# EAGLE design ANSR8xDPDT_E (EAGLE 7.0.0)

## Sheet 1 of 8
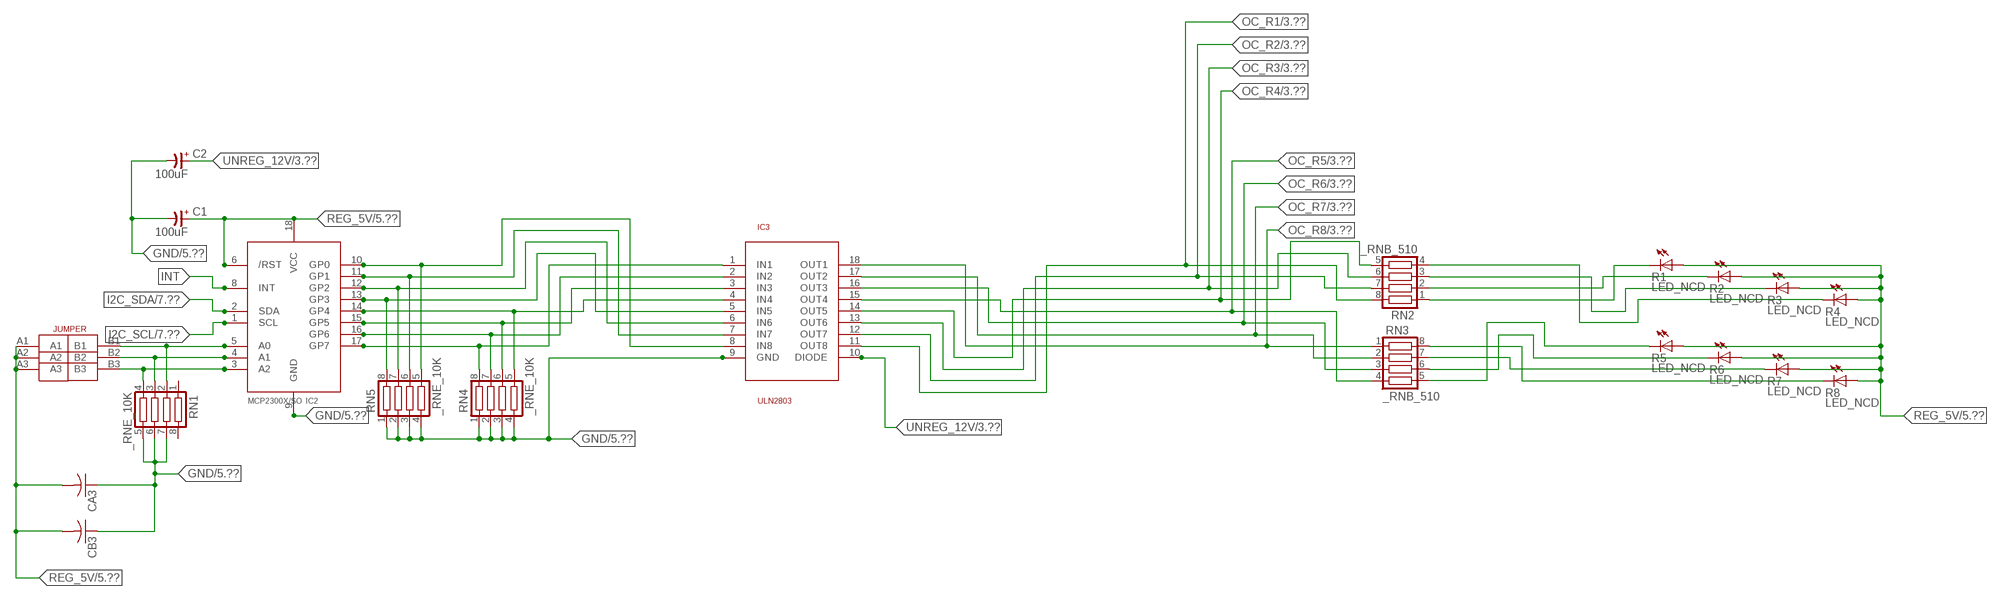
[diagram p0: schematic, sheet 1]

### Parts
C1  100uF  CP-E-025X060  [E-025X060]
C2  100uF  CP-E-025X060  [E-025X060]
CA3  CC1206KRX7R9BB104C1206K  [CC1206KRX7R9BB104]
CB3  TMK316F106ZL-TC1206K  [TMK316F106ZL-T]
IC2  MCP2300X/SO  [SO18W]
IC3  ULN2803  [SO18L]
R1  LED_NCD  [CHIPLED_0603]
R2  LED_NCD  [CHIPLED_0603]
R3  LED_NCD  [CHIPLED_0603]
R4  LED_NCD  [CHIPLED_0603]
R5  LED_NCD  [CHIPLED_0603]
R6  LED_NCD  [CHIPLED_0603]
R7  LED_NCD  [CHIPLED_0603]
R8  LED_NCD  [CHIPLED_0603]
RN1  _RNE_10K  [RNE]
RN2  _RNB_510  [RNB]
RN3  _RNB_510  [RNB]
RN4  _RNE_10K  [RNE]
RN5  _RNE_10K  [RNE]
U$18  JUMPER_3X2  [JUMPER_3X2]

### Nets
GND: C1.- C2.- CA3.1 CB3.1 IC2.9(GND) IC3.9(GND) RN1.5 RN1.6 RN1.7 RN4.1 RN4.2 RN4.3 RN4.4 RN5.1 RN5.2 RN5.3 RN5.4 ; also sheet 5,6,7,8
GP4: IC2.14(GP4) IC3.4(IN4) RN4.5
GP6: IC2.16(GP6) IC3.2(IN2) RN4.7
I2C_SCL: IC2.1(SCL) ; also sheet 7,8
I2C_SDA: IC2.2(SDA) ; also sheet 7,8
INT: IC2.8(INT)
N$6: IC2.5(A0) RN1.2 U$18.B1
N$7: IC2.4(A1) RN1.3 U$18.B2
N$8: IC2.3(A2) RN1.4 U$18.B3
N$20: R1.C RN2.1
N$21: IC2.12(GP2) IC3.6(IN6) RN5.7
N$22: IC2.11(GP1) IC3.7(IN7) RN5.6
N$23: IC2.10(GP0) IC3.8(IN8) RN5.5
N$29: R2.C RN2.2
N$30: R3.C RN2.3
N$31: R4.C RN2.4
N$32: R8.C RN3.8
N$81: R7.C RN3.7
N$82: R6.C RN3.6
N$83: R5.C RN3.5
N$89: IC2.13(GP3) IC3.5(IN5) RN5.8
N$93: IC2.15(GP5) IC3.3(IN3) RN4.6
N$94: IC2.17(GP7) IC3.1(IN1) RN4.8
OC_R1: IC3.11(OUT8) RN2.8 ; also sheet 3
OC_R2: IC3.12(OUT7) RN2.7 ; also sheet 3
OC_R3: IC3.13(OUT6) RN2.6 ; also sheet 3
OC_R4: IC3.14(OUT5) RN2.5 ; also sheet 3
OC_R5: IC3.15(OUT4) RN3.4 ; also sheet 3
OC_R6: IC3.16(OUT3) RN3.3 ; also sheet 3
OC_R7: IC3.17(OUT2) RN3.2 ; also sheet 3
OC_R8: IC3.18(OUT1) RN3.1 ; also sheet 3
REG_5V: C1.+ CA3.2 CB3.2 IC2.6(/RST) IC2.18(VCC) R1.A R2.A R3.A R4.A R5.A R6.A R7.A R8.A U$18.A1 U$18.A2 U$18.A3 ; also sheet 5,6,7,8
UNREG_12V: C2.+ IC3.10(DIODE) ; also sheet 3,5
Unconnected: RN1.1 RN1.8

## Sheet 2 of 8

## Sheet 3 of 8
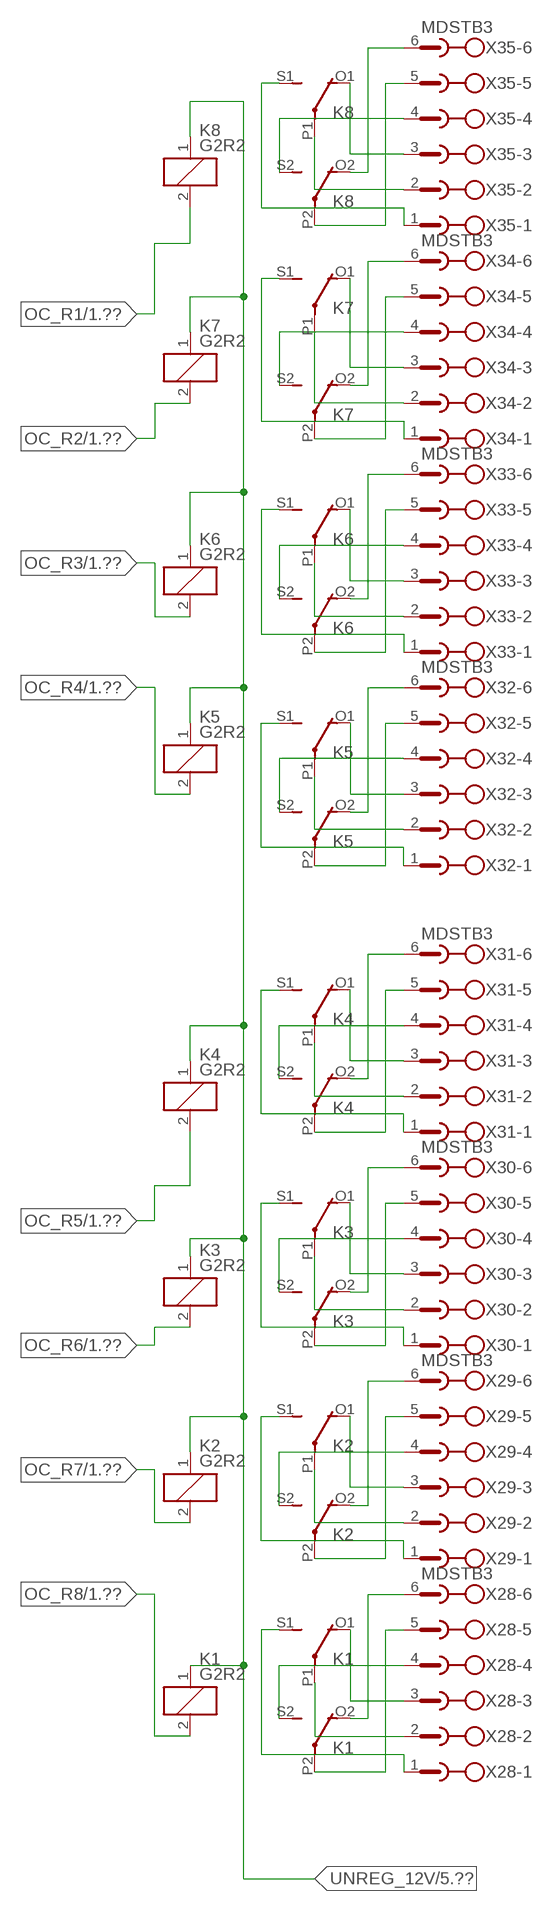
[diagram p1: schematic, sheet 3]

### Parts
K1  G2R2  [G2R2]
K2  G2R2  [G2R2]
K3  G2R2  [G2R2]
K4  G2R2  [G2R2]
K5  G2R2  [G2R2]
K6  G2R2  [G2R2]
K7  G2R2  [G2R2]
K8  G2R2  [G2R2]
X28  MDSTB3  [MDSTB3]
X29  MDSTB3  [MDSTB3]
X30  MDSTB3  [MDSTB3]
X31  MDSTB3  [MDSTB3]
X32  MDSTB3  [MDSTB3]
X33  MDSTB3  [MDSTB3]
X34  MDSTB3  [MDSTB3]
X35  MDSTB3  [MDSTB3]

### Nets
N$84: K1.P2(3:COM) X28.5
N$85: K1.O2(3:NC) X28.6
N$86: K1.S2(3:NO) X28.4
N$87: K1.P1(2:COM) X28.2
N$88: K1.O1(2:NC) X28.3
N$90: K1.S1(2:NO) X28.1
N$91: K2.P2(3:COM) X29.5
N$92: K2.O2(3:NC) X29.6
N$95: K2.S2(3:NO) X29.4
N$96: K2.S1(2:NO) X29.1
N$97: K2.P1(2:COM) X29.2
N$98: K2.O1(2:NC) X29.3
N$99: K3.P2(3:COM) X30.5
N$100: K3.O2(3:NC) X30.6
N$101: K4.P2(3:COM) X31.5
N$102: K4.O2(3:NC) X31.6
N$103: K3.S2(3:NO) X30.4
N$104: K4.S2(3:NO) X31.4
N$105: K3.O1(2:NC) X30.3
N$106: K4.O1(2:NC) X31.3
N$107: K4.P1(2:COM) X31.2
N$108: K3.P1(2:COM) X30.2
N$109: K3.S1(2:NO) X30.1
N$110: K4.S1(2:NO) X31.1
N$111: K5.O2(3:NC) X32.6
N$112: K5.P2(3:COM) X32.5
N$113: K5.S2(3:NO) X32.4
N$114: K5.P1(2:COM) X32.2
N$115: K5.S1(2:NO) X32.1
N$116: K5.O1(2:NC) X32.3
N$117: K6.P2(3:COM) X33.5
N$118: K6.O2(3:NC) X33.6
N$119: K6.P1(2:COM) X33.2
N$120: K6.S1(2:NO) X33.1
N$121: K7.P1(2:COM) X34.2
N$122: K8.P1(2:COM) X35.2
N$316: K8.P2(3:COM) X35.5
N$317: K8.O2(3:NC) X35.6
N$318: K6.O1(2:NC) X33.3
N$319: K8.O1(2:NC) X35.3
N$320: K7.O1(2:NC) X34.3
N$321: K7.O2(3:NC) X34.6
N$322: K7.P2(3:COM) X34.5
N$323: K6.S2(3:NO) X33.4
N$324: K7.S2(3:NO) X34.4
N$325: K7.S1(2:NO) X34.1
N$326: K8.S1(2:NO) X35.1
N$327: K8.S2(3:NO) X35.4
OC_R1: K8.2(1:C2) ; also sheet 1
OC_R2: K7.2(1:C2) ; also sheet 1
OC_R3: K6.2(1:C2) ; also sheet 1
OC_R4: K5.2(1:C2) ; also sheet 1
OC_R5: K4.2(1:C2) ; also sheet 1
OC_R6: K3.2(1:C2) ; also sheet 1
OC_R7: K2.2(1:C2) ; also sheet 1
OC_R8: K1.2(1:C2) ; also sheet 1
UNREG_12V: K1.1(1:C1) K2.1(1:C1) K3.1(1:C1) K4.1(1:C1) K5.1(1:C1) K6.1(1:C1) K7.1(1:C1) K8.1(1:C1) ; also sheet 1,5

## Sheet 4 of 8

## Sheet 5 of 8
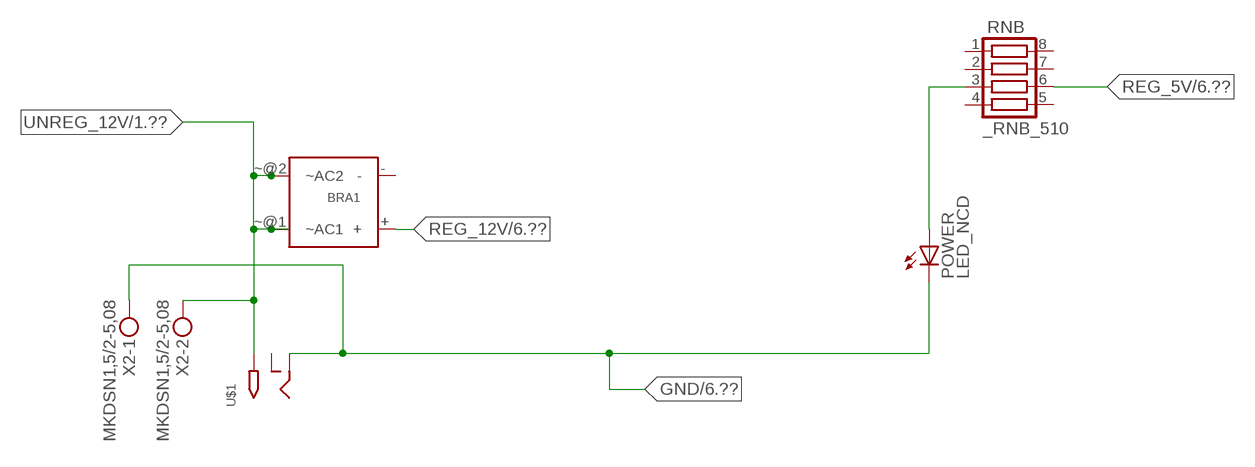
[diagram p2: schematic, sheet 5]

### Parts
BRA1  MB2S_  [MB2S]
POWER  LED_NCD  [CHIPLED_0603]
RNB  _RNB_510  [RNB]
U$1  2.1MMJACK  [PJ-102A]
X2  MKDSN1,5/2-5,08  [MKDSN1,5/2-5,08]

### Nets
GND: POWER.C U$1.RING X2.1 ; also sheet 1,6,7,8
N$2: POWER.A RNB.3
REG_5V: RNB.6 ; also sheet 1,6,7,8
REG_12V: BRA1.+ ; also sheet 6
UNREG_12V: BRA1.~@1(~AC1) BRA1.~@2(~AC2) U$1.TIP X2.2 ; also sheet 1,3
Unconnected: BRA1.- RNB.1 RNB.2 RNB.4 RNB.5 RNB.7 RNB.8 U$1.RING_SW

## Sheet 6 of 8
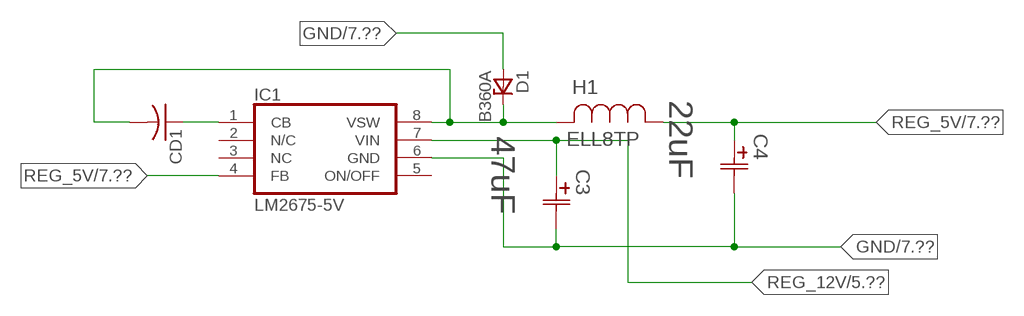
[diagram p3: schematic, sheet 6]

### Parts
C3  47uF  490-5463-6-NDCAP  [C2917(7343)-Y]
C4  22uF  490-5463-6-NDCAP  [C2917(7343)-Y]
CD1  _CD_10NF_50VC1206K  [_CD_10NF_50V]
D1  B360A  [DO214AC_ZENER]
H1  ELL8TP  [IND_ELL8TP]
IC1  LM2675-5V  LM2675  [SO-8]

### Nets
GND: C3.2(C2) C4.2(C2) D1.A IC1.6(GND) ; also sheet 1,5,7,8
N$1: CD1.2 D1.C H1.2 IC1.8(VSW)
N$3: CD1.1 IC1.1(CB)
REG_5V: C4.1(C1) H1.1 IC1.4(FB) ; also sheet 1,5,7,8
REG_12V: C3.1(C1) IC1.7(VIN) ; also sheet 5
Unconnected: IC1.2(N/C) IC1.5(ON/OFF)

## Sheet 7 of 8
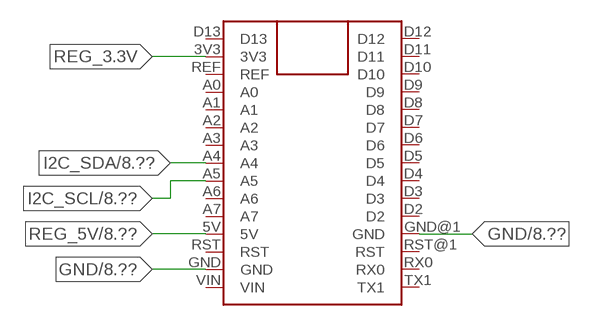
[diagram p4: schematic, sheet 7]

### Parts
FOR_NANO  ARDUINO_NANO  [ARDUINO_NANO]

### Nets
GND: FOR_NANO.GND FOR_NANO.GND@1(GND) ; also sheet 1,5,6,8
I2C_SCL: FOR_NANO.A5 ; also sheet 1,8
I2C_SDA: FOR_NANO.A4 ; also sheet 1,8
REG_3.3V: FOR_NANO.3V3
REG_5V: FOR_NANO.5V ; also sheet 1,5,6,8
Unconnected: FOR_NANO.A0 FOR_NANO.A1 FOR_NANO.A2 FOR_NANO.A3 FOR_NANO.A6 FOR_NANO.A7 FOR_NANO.D2 FOR_NANO.D3 FOR_NANO.D4 FOR_NANO.D5 FOR_NANO.D6 FOR_NANO.D7 FOR_NANO.D8 FOR_NANO.D9 FOR_NANO.D10 FOR_NANO.D11 FOR_NANO.D12 FOR_NANO.D13 FOR_NANO.REF FOR_NANO.RST FOR_NANO.RST@1(RST) FOR_NANO.RX0 FOR_NANO.TX1 FOR_NANO.VIN

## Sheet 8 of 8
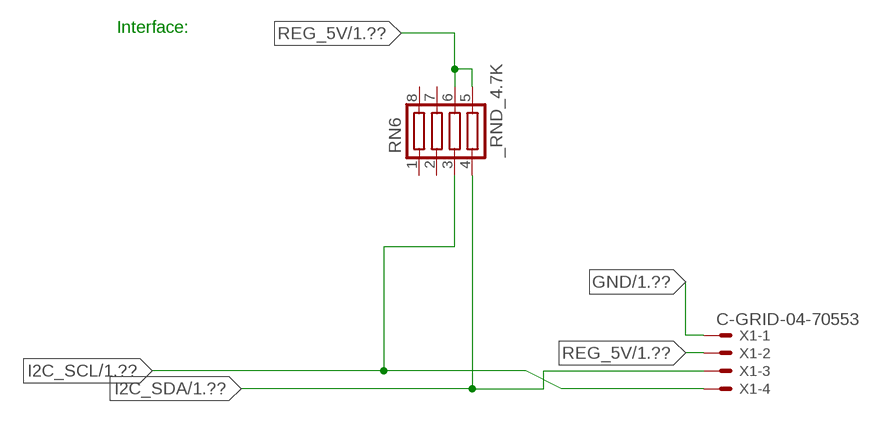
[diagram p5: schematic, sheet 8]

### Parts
RN6  _RND_4.7K  [RND]
X1  C-GRID-04-70553  [70553-04]

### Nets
GND: X1.1 ; also sheet 1,5,6,7
I2C_SCL: RN6.3 X1.4 ; also sheet 1,7
I2C_SDA: RN6.4 X1.3 ; also sheet 1,7
REG_5V: RN6.5 RN6.6 X1.2 ; also sheet 1,5,6,7
Unconnected: RN6.1 RN6.2 RN6.7 RN6.8

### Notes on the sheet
- Interface:

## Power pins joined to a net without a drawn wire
NC: IC1.3(NC)

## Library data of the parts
BRA1 = NCD_ULTIMATE_LIBRARY:MB2S: Bridge Rectifier BRA MB2S 200V 500ma Digikey MB2S-TPMSTR-ND/MB2S-TP
C1 C2 = NCD_ULTIMATE_LIBRARY:CP-: Capacitors All Kinds POLARIZED CAP
C3 C4 = NCD_ULTIMATE_bhaskar:490-5463-6-ND: NCD CAP
CA3 = NCD_ULTIMATE_LIBRARY:CC1206KRX7R9BB104: Capacitor CA .1uF 50V SMT C1206K CC1206KRX7R9BB104
CB3 = NCD_ULTIMATE_LIBRARY:TMK316F106ZL-T: Capacitor CB 10uF SMT 1206 TMK316F106ZL-T
CD1 = NCD_ULTIMATE_LIBRARY:_CD_10NF_50V: Capacitor 10nF SMT
D1 = NCD_ULTIMATE_bhaskar:B360A: NCD DIODE B350A/B360A
FOR_NANO = NCD_ULTIMATE_CONNECTORS:ARDUINO_NANO
H1 = NCD_ULTIMATE_bhaskar:ELL8TP: NCD coil
IC1 = NCD_ULTIMATE_bhaskar:LM2675: LM2675 NCD http://www.ti.com/lit/ds/symlink/lm2675.pdf
IC2 = NCD_ULTIMATE_LIBRARY:MCP2300X: Semiconductor Port Expander I/O 8-Bit I2C MCP23008 Inexpensive i2c i/o expander - 8 general purpose i/o pins with optional pullups
IC3 = NCD_ULTIMATE_LIBRARY:ULN2803: Semiconductor 8 O.C. N-Channel Transistor Driver Digikey ULN2803AFWGCELTR-ND/ULN2803AFWG,C,EL
K1-K8 = NCD_ULTIMATE_LIBRARY:G2R2: RELAY 2 x switch, Omron
POWER = NCD_ULTIMATE_bhaskar:LED_NCD
R1-R8 = NCD_ULTIMATE_LIBRARY:LED_NCD: LED Digikey 754-1132-2-ND/APT2012SRCPRV
RN1 RN4 RN5 = NCD_ULTIMATE_LIBRARY:_RNE_10K: Resistor Array RNE SMT 10K x 4 Single Resistor Source: http://www.ctscorp.com/components/Datasheets/CTSChipArrayDs.pdf Digikey 742C083103JPTR-ND/742C083103JP; OC_FARNELL: unknown; OC_NEWARK: unknown
RN2 RN3 RNB = NCD_ULTIMATE_LIBRARY:_RNB_510: Resistor Array RNB SMT 510 x 4 Single Resistor Source: http://www.ctscorp.com/components/Datasheets/CTSChipArrayDs.pdf Digikey 742C083511JPTR-ND/ 742C083511JP; OC_FARNELL: unknown; OC_NEWARK: unknown
RN6 = NCD_ULTIMATE_LIBRARY:_RND_4.7K: Resistor Array RND SMT 4.7K x 4 Single Resistor Source: http://www.ctscorp.com/components/Datasheets/CTSChipArrayDs.pdf Digikey 742C083472JPTR-ND/742C083472JP; OC_FARNELL: unknown; OC_NEWARK: unknown
U$1 = NCD_ULTIMATE_CONNECTORS:2.1MMJACK: 2.1mm x 5.5mm DC jack with internal switch. Digikey part #PJ-102A, 4UCON part #05537 By microbuilder.eu
U$18 = NCD_ULTIMATE_CONNECTORS:JUMPER_3X2
X1 = NCD_ULTIMATE_CONNECTORS:C-GRID-04: CONNECTOR 4-Pos I2C wire to board 2.54 mm (0.100") pitch header Digikey WM1342-ND/0015912045; OC_FARNELL: unknown; OC_NEWARK: unknown
X2 = NCD_ULTIMATE_CONNECTORS:MKDSN1,5/2-5,08: MKDSN 1,5/ 2-5,08 Printklemme
X28-X35 = NCD_ULTIMATE_LIBRARY:MDSTB3: PHOENIX

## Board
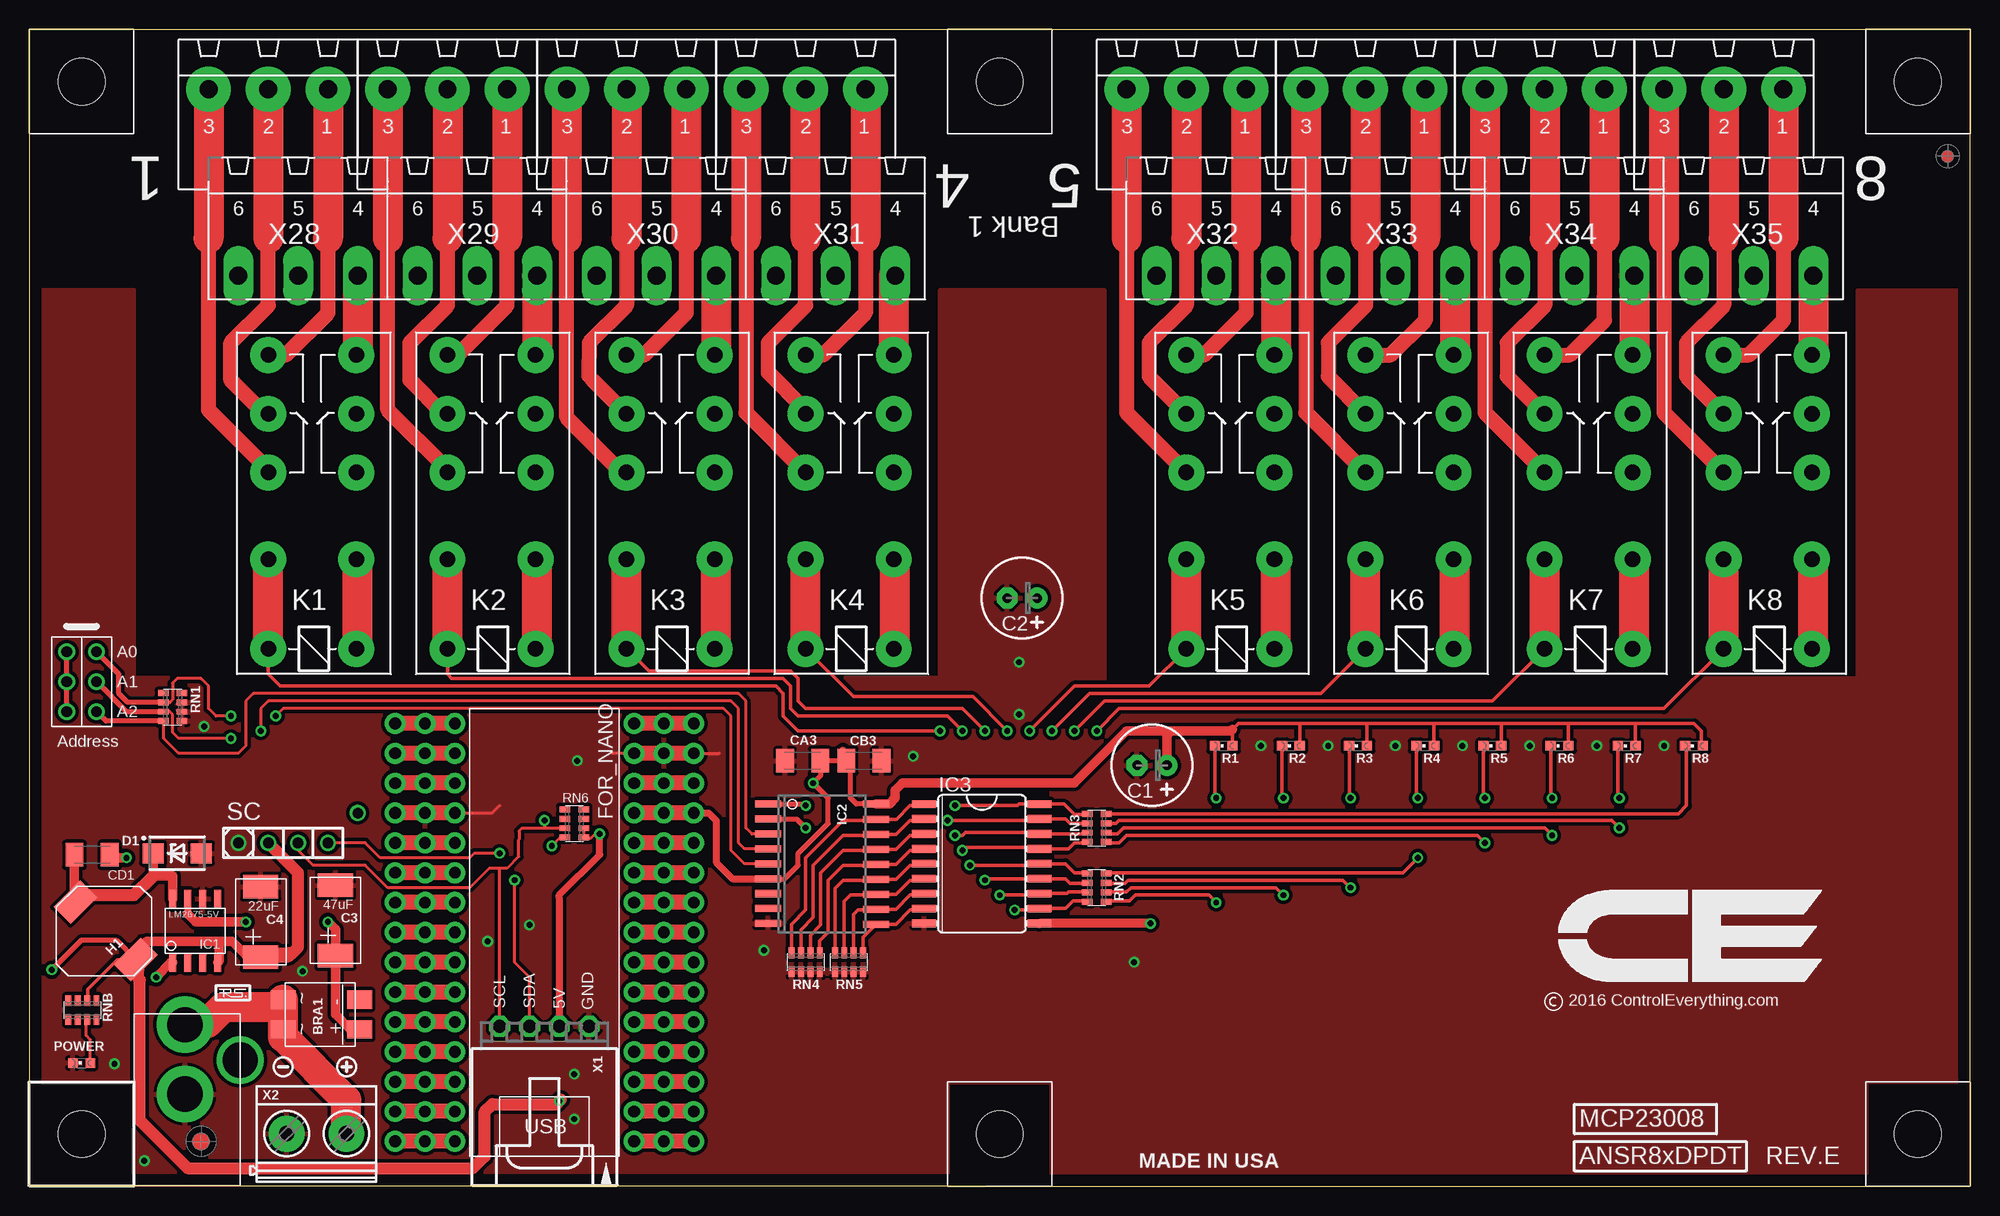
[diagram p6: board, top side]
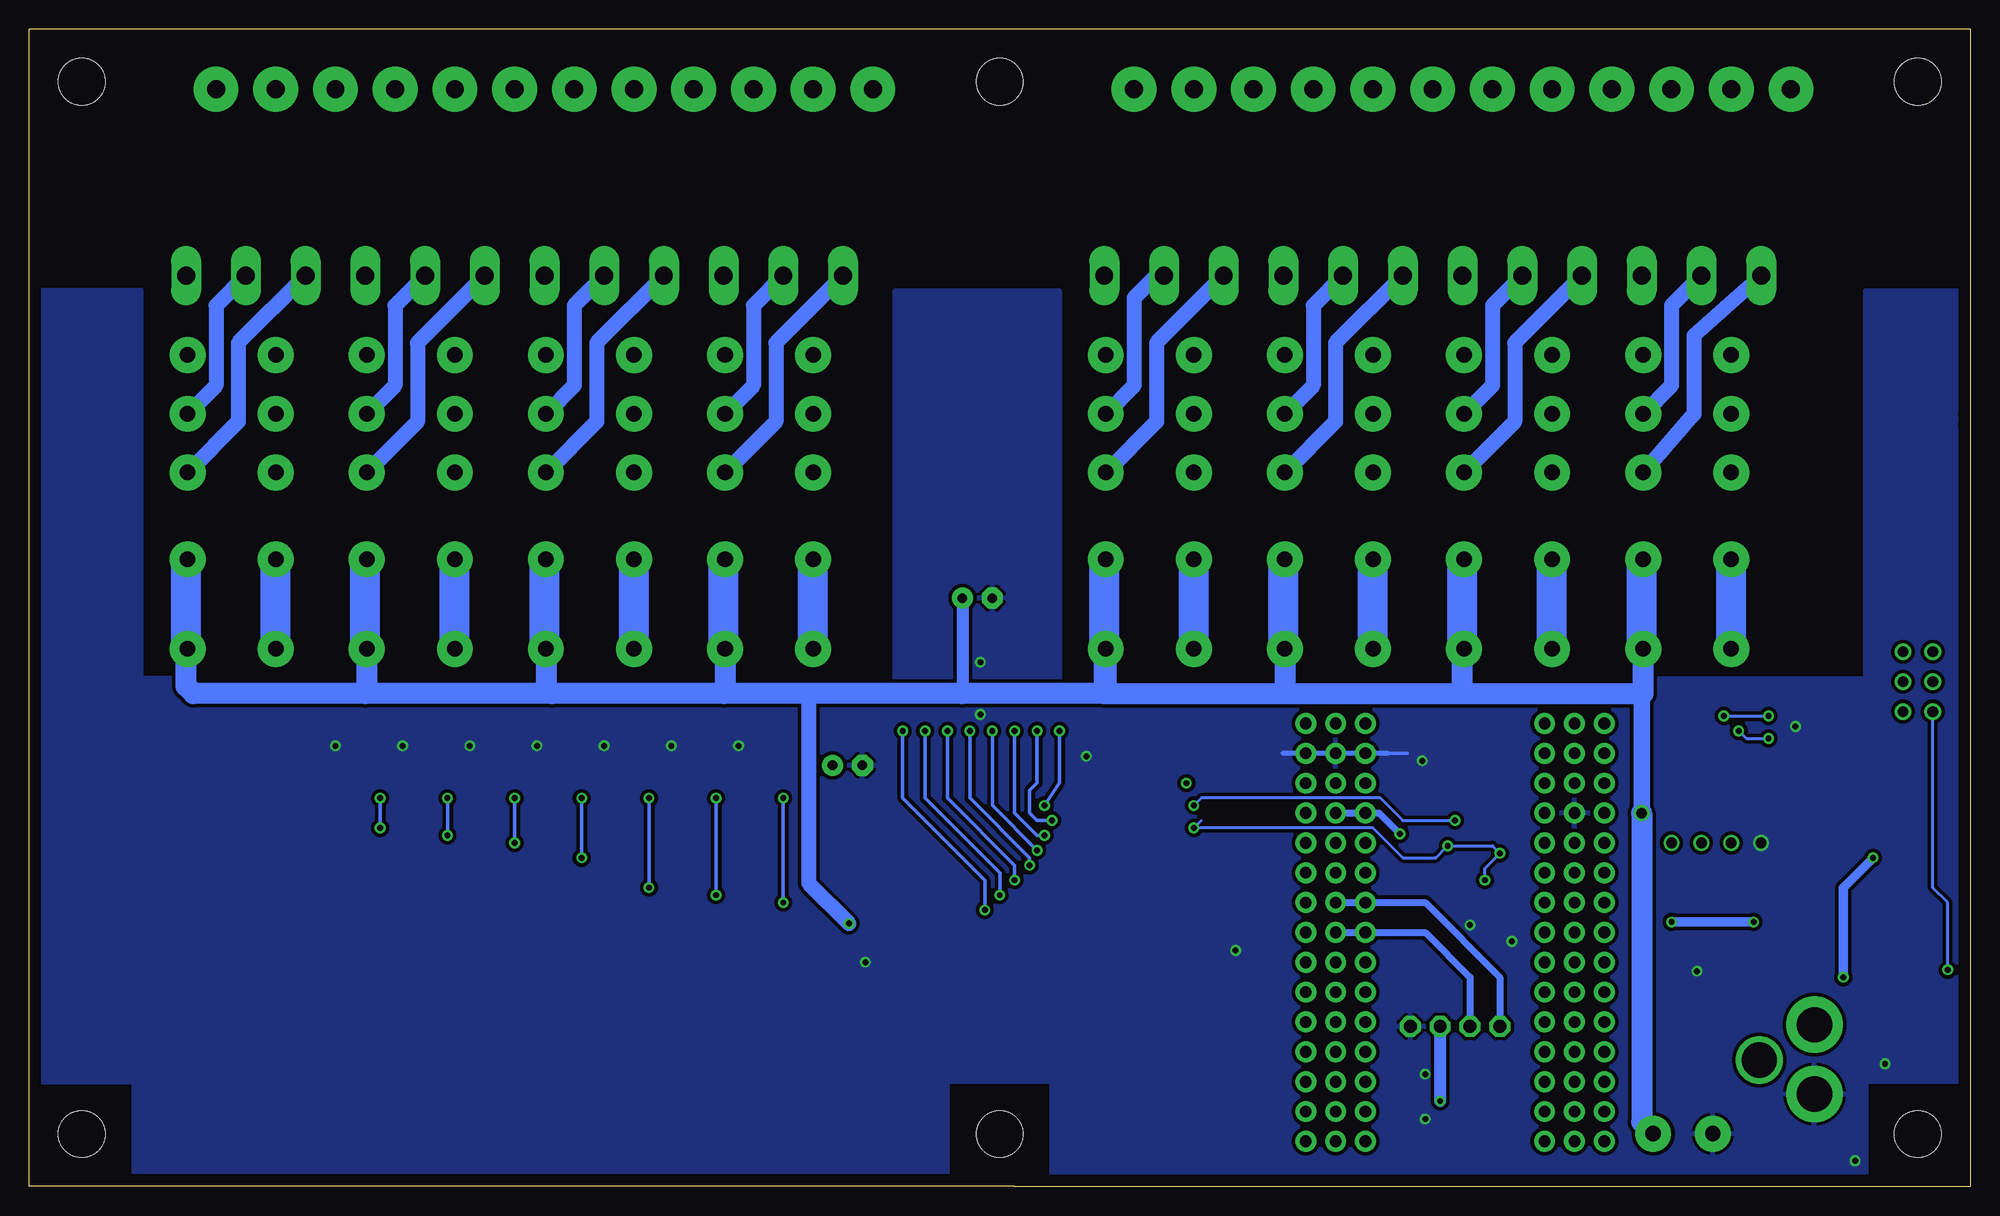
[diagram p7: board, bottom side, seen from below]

Size 165.1 x 98.42 mm. Coordinates in mm from the lower left corner, seen from the top.
Outline: 81.28,0 82.53,0
Outline: 0,65.71 0,64.77
Outline: 0,64.77 0,0 81.28,0
Outline: 81.28,0 165.1,0 165.1,98.42 0,98.42 0,64.77
Copper layers (1*16): Top 0.035mm / dielectric 1.5mm / Bottom 0.035mm
Design rules "default": minimum track width 10mil, minimum drill 24mil, track to track 8mil, track to pad 8mil, pad to pad 8mil, via to via 8mil, smd to smd 8mil, copper to edge 40mil, drill to drill 8mil, minimum pad ring 10mil, minimum via ring 8mil, stop-mask expansion 4mil, vias tented up to drill 0mil, thermal gap 10mil
Holes 3.96 mm at 4.45,4.45 4.45,4.45 4.45,4.45 4.45,4.45

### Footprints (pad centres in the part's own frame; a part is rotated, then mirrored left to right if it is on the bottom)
MB2S = smd 1.55 x 2.1: + 0,-6.5; - 2.54,-6.5; ~@1 0,0; ~@2 2.54,0
E-025X060 = drill 0.813 pad 1.778: + -1.27,0 | drill 0.813 pad 1.778 octagon: - 1.27,0
C2917(7343)-Y = smd 2 x 3: 1 -3,0; 2 3,0
CC1206KRX7R9BB104 = smd 1.5 x 2: 1 -1.5,0; 2 1.5,0
TMK316F106ZL-T = smd 1.5 x 2: 1 -1.5,0; 2 1.5,0
_CD_10NF_50V = smd 1.5 x 2: 1 -1.5,0; 2 1.5,0
DO214AC_ZENER = smd 1.8 x 1.7: A 2.05,0; C -2.05,0
ARDUINO_NANO = drill 1 pad 1.778: 3V1 -2.54,-2.54; 3V3 0,-2.54; 5V 0,-27.94; 5V1 -2.54,-27.94; A0 0,-7.62; A1 0,-10.16; A2 0,-12.7; A3 0,-15.24; A4 0,-17.78; A5 0,-20.32; A6 0,-22.86; A7 0,-25.4; A8 -2.54,-7.62; A9 -2.54,-10.16; A10 -2.54,-12.7; A11 -2.54,-15.24; A12 -2.54,-17.78; A13 -2.54,-20.32; A14 -2.54,-22.86; A15 -2.54,-25.4; D1 -2.54,0; D2 20.32,-25.4; D3 20.32,-22.86; D4 20.32,-20.32; D5 20.32,-17.78; D6 20.32,-15.24; D7 20.32,-12.7; D8 20.32,-10.16; D9 20.32,-7.62; D10 20.32,-5.08; D11 20.32,-2.54; D12 20.32,0; D13 0,0; D14 22.86,0; D15 22.86,-2.54; D16 22.86,-5.08; D17 22.86,-7.62; D18 22.86,-10.16; D19 22.86,-12.7; D20 22.86,-15.24; D21 22.86,-17.78; D22 22.86,-20.32; D23 22.86,-22.86; D24 22.86,-25.4; GND 0,-33.02; GND1 -2.54,-33.02; GND@1 20.32,-27.94; GND@2 22.86,-27.94; P$16 2.54,0; P$17 2.54,-2.54; P$18 2.54,-5.08; P$19 2.54,-7.62; P$20 2.54,-10.16; P$21 2.54,-12.7; P$22 2.54,-15.24; P$23 2.54,-17.78; P$24 2.54,-20.32; P$25 2.54,-22.86; P$26 2.54,-25.4; P$27 2.54,-27.94; P$28 2.54,-30.48; P$29 2.54,-33.02; P$30 2.54,-35.56; P$31 17.78,0; P$32 17.78,-2.54; P$33 17.78,-5.08; P$34 17.78,-7.62; P$35 17.78,-10.16; P$36 17.78,-12.7; P$37 17.78,-15.24; P$38 17.78,-17.78; P$39 17.78,-20.32; P$40 17.78,-22.86; P$41 17.78,-25.4; P$42 17.78,-27.94; P$43 17.78,-30.48; P$44 17.78,-33.02; P$45 17.78,-35.56; REF 0,-5.08; REF1 -2.54,-5.08; RST 0,-30.48; RST1 -2.54,-30.48; RST@1 20.32,-30.48; RST@2 22.86,-30.48; RX0 20.32,-33.02; RX1 22.86,-33.02; TX1 20.32,-35.56; TX2 22.86,-35.56; VIN 0,-35.56; VIN1 -2.54,-35.56
IND_ELL8TP = smd 2.054 x 3.2 rotated 45: 1 -2.442,-2.696; 2 2.442,2.442
SO-8 = smd 0.6 x 1.55: 1 -1.905,-2.69; 2 -0.635,-2.69; 3 0.635,-2.69; 4 1.905,-2.69; 5 1.905,2.71; 6 0.635,2.71; 7 -0.635,2.71; 8 -1.905,2.71
SO18W = smd 0.6 x 2.2: 1 -4.445,-4.6; 2 -3.175,-4.6; 3 -1.905,-4.6; 4 -0.635,-4.6; 5 0.635,-4.6; 6 1.905,-4.6; 7 3.175,-4.6; 8 4.445,-4.6; 9 5.715,-4.6; 10 5.775,4.6; 11 4.505,4.6; 12 3.235,4.6; 13 1.965,4.6; 14 0.695,4.6; 15 -0.575,4.6; 16 -1.845,4.6; 17 -3.145,4.6; 18 -4.445,4.6
SO18L = smd 0.66 x 2.032: 1 -5.08,-4.902; 2 -3.81,-4.902; 3 -2.54,-4.902; 4 -1.27,-4.902; 5 0,-4.902; 6 1.27,-4.902; 7 2.54,-4.902; 8 3.81,-4.902; 9 5.08,-4.902; 10 5.08,4.902; 11 3.81,4.902; 12 2.54,4.902; 13 1.27,4.902; 14 0,4.902; 15 -1.27,4.902; 16 -2.54,4.902; 17 -3.81,4.902; 18 -5.08,4.902
G2R2 = drill 1.321 pad 3.048: 1 -2.54,-3.683; 2 -2.54,3.81; 3 5.08,-3.683; 4 5.08,3.81; O1 12.471,3.81; O2 12.471,-3.683; P1 17.45,3.81; P2 17.45,-3.683; S1 22.454,3.81; S2 22.454,-3.683
CHIPLED_0603 = smd 0.8 x 0.8: A 0,-0.75; C 0,0.75
CHIPLED_0603' = smd 0.8 x 0.876: A 0,-0.75; C 0,0.75
RNE = smd 0.5 x 0.9: 1 -1.2,-0.8; 2 -0.4,-0.8; 3 0.4,-0.8; 4 1.2,-0.8; 5 1.2,0.8; 6 0.4,0.8; 7 -0.4,0.8; 8 -1.2,0.8
RNB = smd 0.5 x 0.9: 1 -1.2,-0.8; 2 -0.4,-0.8; 3 0.4,-0.8; 4 1.2,-0.8; 5 1.2,0.8; 6 0.4,0.8; 7 -0.4,0.8; 8 -1.2,0.8
RND = smd 0.5 x 0.9: 1 -1.2,-0.8; 2 -0.4,-0.8; 3 0.4,-0.8; 4 1.2,-0.8; 5 1.2,0.8; 6 0.4,0.8; 7 -0.4,0.8; 8 -1.2,0.8
PJ-102A = drill 3 pad 4.8: RING 0.1,-3.39; TIP 0.1,-9.29 | drill 3 pad 3.251: RING_SW -4.6,-6.29
PCB_MOUNTING_HOLE = hole 3.962: 4.445,4.445
JUMPER_3X2 = drill 0.9: A1 0,5.08; A2 0,2.54; A3 0,0; B1 2.54,5.08; B2 2.54,2.54; B3 2.54,0
70553-04 = drill 1.1 pad 1.778 octagon: 1 -3.81,-7.62; 2 -1.27,-7.62; 3 1.27,-7.62; 4 3.81,-7.62
MKDSN1,5/2-5,08 = drill 1.3 pad 3.048: 1 -2.561,0.025; 2 2.519,0.025
MDSTB3 = drill 1.524 pad 3.81: 1 -3.81,-10.795; 2 1.27,-10.795; 3 6.35,-10.795 | drill 1.524 pad 2.54 long: 4 -6.35,5.08; 5 -1.27,5.08; 6 3.81,5.08

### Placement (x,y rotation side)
BRA1  21.59,13.34 90 top
C1  95.5,35.81 180 top
C2  84.45,50.04 180 top
C3  26.04,22.61 90 top
C4  19.68,22.48 90 top
CA3  65.79,36.2 0 top
CB3  70.99,36.2 180 top
CD1  5.33,28.19 180 top
D1  12.57,28.32 0 top
FOR_NANO  53.98,3.81 180 top
H1  6.35,21.72 90 top
IC1  14.1,21.72 0 top
IC2  67.44,28.07 270 top
IC3  81.03,27.43 270 top
K1  24.13,48.26 90 top
K2  39.37,48.26 90 top
K3  54.61,48.26 90 top
K4  69.85,48.26 90 top
K5  102.23,48.26 90 top
K6  117.47,48.26 90 top
K7  132.72,48.26 90 top
K8  147.96,48.26 90 top
POWER  4.45,10.48 90 top
R1  LED_NCD  [CHIPLED_0603']  101.6,37.47 90 top
R2  LED_NCD  [CHIPLED_0603']  107.31,37.47 90 top
R3  LED_NCD  [CHIPLED_0603']  113.03,37.47 90 top
R4  LED_NCD  [CHIPLED_0603']  118.75,37.47 90 top
R5  LED_NCD  [CHIPLED_0603']  124.46,37.47 90 top
R6  LED_NCD  [CHIPLED_0603']  130.18,37.47 90 top
R7  LED_NCD  [CHIPLED_0603']  135.89,37.47 90 top
R8  LED_NCD  [CHIPLED_0603']  141.6,37.47 90 top
RN1  12.19,40.77 270 top
RN2  90.81,25.4 90 top
RN3  90.81,30.48 270 top
RN4  66.04,19.05 0 top
RN5  69.72,19.05 0 top
RN6  46.35,30.86 270 top
RNB  4.51,14.99 0 top
U$1  13.34,4.45 180 top
U$2  [VISION_REF15]  14.61,3.81 0 top
U$3  [ICON_MINUS]  21.59,10.16 180 top
U$5  [ICON_PLUS]  26.99,10.16 90 top
U$6  PCB_MOUNTING_HOLE  [PCB_MOUNTING_HOLE]  87,0 90 top
U$9  PCB_MOUNTING_HOLE  [PCB_MOUNTING_HOLE]  87,89.53 90 top
U$11  PCB_MOUNTING_HOLE  [PCB_MOUNTING_HOLE]  165.1,0 90 top
U$13  PCB_MOUNTING_HOLE  [PCB_MOUNTING_HOLE]  8.89,89.53 90 top
U$14  PCB_MOUNTING_HOLE  [PCB_MOUNTING_HOLE]  165.1,89.53 90 top
U$16  [VISION_REF10]  163.19,87.63 270 top
U$18  3.17,40.39 0 top
U$21  [ICON_USA]  94.36,1.52 0 top
X1  43.81,5.97 180 top
X2  24.45,4.45 0 top
X28  21.59,82.55 180 top
X29  36.83,82.55 180 top
X30  52.07,82.55 180 top
X31  67.31,82.55 180 top
X32  99.69,82.55 180 top
X33  114.94,82.55 180 top
X34  130.18,82.55 180 top
X35  145.41,82.55 180 top

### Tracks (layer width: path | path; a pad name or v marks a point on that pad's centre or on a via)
GND  (via drill 0.5, 0.9)
  Top 0.254: 36.2,31.75 39.37,31.75 40.01,32.39 | FOR_NANO.GND@1 32.38,31.75 | 49.53,36.83 56.52,36.83 58.67,36.83
  Top 1.016: X1.1 47.62,13.74
  Bottom 0.254: 51.44,36.83 FOR_NANO.GND
  Bottom 0.305: 47.88,36.83 49.53,36.83 51.44,36.83
  Bottom 0.406: 49.53,36.83 58.42,36.83
  other vias: 14.86,39.12 62.48,20.07 127.64,37.47 93.98,19.05 133.35,37.47 139.06,37.47 121.92,37.47 116.2,37.47 110.49,37.47 104.78,37.47 75.18,36.58 84.2,40.13 84.2,44.58 9.78,2.16 17.78,29.21 46.35,9.53 46.61,36.2 46.35,5.72 42.55,22.23 38.99,20.83 7.24,10.41 23.24,18.29
  pour Bottom (isolate 0.305): -1.27,8.89 8.89,8.89 8.89,0 78.11,0 78.11,8.89 91.44,8.89 91.44,76.2 77.47,76.2 77.47,43.18 8.89,43.18 8.89,76.2 -1.27,76.2
  pour Top (isolate 0.305): -3.17,8.89 8.89,8.89 8.89,0 78.11,0 78.11,8.89 91.44,8.89 91.44,76.2 77.47,76.2 77.47,43.18 8.89,43.18 8.89,76.2 -3.17,76.2
  pour Top (isolate 0.305): 87,43.18 155.57,43.18 155.57,76.2 168.28,76.2 168.28,8.89 156.21,8.89 156.21,0 87,0
  pour Bottom (isolate 0.305): 87,0 87,43.18 155.57,43.18 155.57,76.2 170.81,76.2 170.81,8.89 156.21,8.89 156.21,0
GP4
  Top 0.305: RN4.5 67.24,20.88 67.94,21.59 67.94,26.04 69.22,27.3 71.97,27.3 IC2.14 73.73,27.37 74.93,28.57 76,28.57 IC3.4
GP6
  Top 0.305: RN4.7 65.64,21.83 66.67,22.86 66.67,27.3 69.22,29.84 71.97,29.84 IC2.16 73.73,29.91 74.93,31.12 76,31.12 IC3.2
I2C_SCL  (via drill 0.5, 0.9)
  Top 0.254: 40.01,27.05 40.64,27.05 41.64,28.05 41.64,29.48 41.66,29.5 41.66,30.23 41.89,30.46 RN6.3 45.54,30.48 43.81,30.48 v43.81,31.12 | 40.01,27.05 39.12,27.05 37.47,25.4 30.48,25.4 28.57,27.3 24.13,27.3 22.86,28.57 v22.86,29.21 | X1.4 40.01,27.05
  Top 0.406: IC2.1 65.91,32.51 v66.04,32.39
  Bottom 0.254: v43.81,31.12 48.26,31.12 50.16,33.02 65.41,33.02 v66.04,32.39
  Bottom 0.61: FOR_NANO.A5 46.35,24.13 40.01,17.78 X1.4
I2C_SDA  (via drill 0.5, 0.9)
  Top 0.254: RN6.4 45.16,29.66 v44.45,28.96 | 40,28.33 v40.01,28.32 37.85,28.32 37.47,27.94 29.84,27.94 28.57,29.21 v25.4,29.21 | X1.3 42.55,17.78 41.27,19.05 v41.27,26.04
  Top 0.406: IC2.2 65.28,31.24 v66.04,30.48
  Bottom 0.254: 65.41,31.12 v66.04,30.48 50.8,30.48 48.26,27.94 45.47,27.94 v44.45,28.96 40.64,28.96 v40.01,28.32 41.27,27.05 v41.27,26.04
  Bottom 0.61: FOR_NANO.A4 46.35,21.59 42.55,17.78 X1.3
N$1
  Top 0.813: H1.2 3.88,24.77 | D1.C 10.52,26.4 12.19,26.38 IC1.8 | CD1.2 3.83,24.15 4.45,24.77
  Top 1.016: 3.88,24.77 4.45,24.77 8.89,24.77 10.52,26.4
N$2
  Top 0.254: POWER.A 5.2,12.46 4.83,12.83 4.83,14.1 RNB.3
  Top 0.406: 4.95,14.14 RNB.3
N$3  (via drill 0.5)
  Top 0.813: IC1.1 12.04,19.03 v10.79,17.78 | v8.26,27.94 7.72,27.94 CD1.1
  Bottom 0.813: v10.79,17.78 10.79,25.4 v8.26,27.94
N$6  (via drill 0.5)
  Top 0.254: IC2.5 60.83,27.43 59.69,28.57 59.69,40 59.05,40.64 21.59,40.64 v20.95,40 | v17.14,40 15.88,40 15.24,40.64 15.24,42.55 14.61,43.18 12.57,43.18 12.19,42.8 12.19,41.4 11.94,41.15 11.41,41.15 RN1.2
  Top 0.406: RN1.2 8.36,41.17 7.62,41.91 7.62,43.56 U$18.B1
  Bottom 0.254: v20.95,40 v17.14,40
N$7  (via drill 0.5)
  Top 0.254: IC2.4 60.83,28.7 60.33,29.21 60.33,40.64 59.69,41.27 20.32,41.27 19.68,40.64 v19.68,38.73 | v17.14,38.1 12.7,38.1 12.19,38.61 12.19,40.13 11.94,40.39 11.41,40.39 RN1.3
  Top 0.406: RN1.3 8.27,40.37 U$18.B2
  Bottom 0.254: v19.68,38.73 19.05,38.1 v17.14,38.1
N$8
  Top 0.254: IC2.3 61.47,29.97 60.96,30.48 60.96,41.27 60.33,41.91 19.05,41.91 18.41,41.27 18.41,37.47 17.78,36.83 12.7,36.83 11.43,38.1 11.43,39.53 RN1.4
  Top 0.406: RN1.4 6.53,39.57 U$18.B3
N$20  (via drill 0.5)
  Top 0.305: R1.C 100.85,33.14 v100.97,33.02 | v100.97,24.13 100.33,24.77 94.11,24.77 93.6,24.26 91.66,24.26 RN2.1
  Bottom 0.305: v100.97,33.02 v100.97,24.13
N$21
  Top 0.305: RN5.7 69.32,24.24 69.85,24.77 71.97,24.77 IC2.12 73.73,24.83 74.93,26.04 76,26.04 IC3.6
N$22
  Top 0.305: RN5.6 70.12,23.13 70.48,23.5 71.97,23.5 IC2.11 73.73,23.56 74.93,24.77 76,24.77 IC3.7
N$23
  Top 0.254: 71.97,22.23 IC2.10
  Top 0.305: RN5.5 70.92,21.18 IC2.10 73.73,22.29 74.93,23.5 76,23.5 IC3.8
N$29  (via drill 0.5)
  Top 0.305: R2.C 106.56,33.14 v106.68,33.02 | v106.68,24.77 106.05,25.4 93.73,25.4 93.34,25.02 91.62,25.02 RN2.2
  Bottom 0.305: v106.68,33.02 v106.68,24.77
N$30  (via drill 0.5)
  Top 0.305: R3.C 112.28,33.14 v112.39,33.02 | v112.39,25.4 111.76,26.04 93.47,26.04 93.22,25.78 91.62,25.78 RN2.3
  Bottom 0.305: v112.39,33.02 v112.39,25.4
N$31  (via drill 0.5)
  Top 0.305: R4.C 118,33.14 v118.11,33.02 | v118.11,27.94 116.84,26.67 91.67,26.67 RN2.4
  Bottom 0.305: v118.11,33.02 v118.11,27.94
N$32
  Top 0.305: RN3.8 140.26,31.68 140.97,32.39 140.97,37.35 R8.C
N$81  (via drill 0.5)
  Top 0.305: R7.C 135.14,33.14 v135.25,33.02 | v135.25,30.48 134.62,31.12 92.71,31.12 92.46,30.86 91.62,30.86 RN3.7
  Bottom 0.305: v135.25,33.02 v135.25,30.48
N$82  (via drill 0.5)
  Top 0.305: R6.C 129.43,33.14 v129.54,33.02 | v129.54,29.84 128.91,30.48 93.09,30.48 92.58,29.97 91.71,29.97 RN3.6
  Bottom 0.305: v129.54,33.02 v129.54,29.84
N$83  (via drill 0.5)
  Top 0.305: R5.C 123.71,33.14 v123.83,33.02 | v123.83,29.21 123.19,29.84 93.34,29.84 92.71,29.21 91.67,29.21 RN3.5
  Bottom 0.305: v123.83,33.02 v123.83,29.21
N$84
  Bottom 1.27: X28.5 25.4,74.93 25.4,68.12 K1.P2
N$85
  Bottom 1.27: X28.6 23.5,72.39 23.5,65.68 K1.O2
N$86
  Top 2.54: X28.4 27.94,70.84 K1.S2
N$87
  Top 1.27: K1.P1 20.02,65.71 17.14,68.58 17.14,71.75 20.32,74.93 20.32,80.64
  Top 2.54: X28.2 20.32,80.64
N$88
  Top 1.27: K1.O1 20.32,60.96 15.24,66.04 15.24,80.64
  Top 2.54: X28.3 15.24,80.64
N$89
  Top 0.305: RN5.8 68.52,25.34 69.22,26.04 71.97,26.04 IC2.13 73.73,26.1 74.93,27.3 76,27.3 IC3.5
N$90
  Top 1.27: 25.4,80.64 25.4,74.3 21.82,70.71 K1.S1
  Top 2.54: X28.1 25.4,80.64
N$91
  Bottom 1.27: X29.5 40.64,74.93 40.64,68.12 K2.P2
N$92
  Bottom 1.27: X29.6 38.73,71.75 38.73,65.05 K2.O2
N$93
  Top 0.305: RN4.6 66.44,21.36 67.31,22.23 67.31,26.67 69.22,28.57 71.97,28.57 IC2.15 73.73,28.64 74.93,29.84 76,29.84 IC3.3
N$94
  Top 0.305: RN4.8 64.84,22.3 66.04,23.5 66.04,27.94 69.22,31.12 71.94,31.12 IC2.17 73.76,31.21 74.93,32.39 76,32.39 IC3.1
N$95
  Top 2.54: X29.4 43.18,70.84 K2.S2
N$96
  Top 1.27: 40.64,80.64 40.64,74.93 36.42,70.71 K2.S1
  Top 2.54: X29.1 40.64,80.64
N$97
  Top 1.27: K2.P1 35.26,65.71 32.38,68.58 32.38,71.75 35.56,74.93 35.56,80.64
  Top 2.54: X29.2 35.56,80.64
N$98
  Top 1.27: K2.O1 35.56,60.96 30.48,66.04 30.48,80.64
  Top 2.54: X29.3 30.48,80.64
N$99
  Bottom 1.27: X30.5 55.88,74.93 55.88,68.12 K3.P2
N$100
  Bottom 1.27: X30.6 53.98,71.75 53.98,65.05 K3.O2
N$101
  Bottom 1.27: X31.5 69.22,77.47 71.12,75.56 71.12,68.12 K4.P2
N$102
  Bottom 1.27: X31.6 69.22,71.75 69.22,65.05 K4.O2
N$103
  Top 2.54: X30.4 58.42,70.84 K3.S2
N$104
  Top 2.54: X31.4 73.53,77.47 K4.S2
N$105
  Top 1.27: K3.O1 50.39,60.73 45.72,65.41 45.72,80.64
  Top 2.54: X30.3 45.72,80.64
N$106
  Top 1.27: 60.96,80.64 60.96,65.81 K4.O1
  Top 2.54: X31.3 60.96,80.64
N$107
  Top 1.27: K4.P1 66.04,66.04 62.87,69.22 62.87,71.75 66.04,74.93 66.04,80.64
  Top 2.54: 66.04,80.64 X31.2
N$108
  Top 1.27: 50.8,80.64 50.8,74.93 47.62,71.75 47.57,68.96 47.93,68.58 K3.P1
  Top 2.54: X30.2 50.8,80.64
N$109
  Top 1.27: 55.88,80.64 55.88,74.3 52.3,70.71 K3.S1
  Top 2.54: X30.1 55.88,80.64
N$110
  Top 1.27: 71.12,80.64 71.12,74.3 67.54,70.71 K4.S1
  Top 2.54: X31.1 71.12,80.64
N$111
  Bottom 1.27: X32.6 101.6,71.75 101.6,65.05 K5.O2
N$112
  Bottom 1.27: X32.5 103.5,74.93 103.5,68.12 K5.P2
N$113
  Top 2.54: X32.4 106.05,70.84 K5.S2
N$114
  Top 1.27: 98.42,80.64 98.42,74.93 95.25,71.75 95.25,68.88 K5.P1
  Top 2.54: X32.2 98.42,80.64
N$115
  Top 1.27: 103.5,80.64 103.5,74.3 99.92,70.71 K5.S1
  Top 2.54: X32.1 103.5,80.64
N$116
  Top 1.27: 93.34,80.64 93.34,65.81 K5.O1
  Top 2.54: X32.3 93.34,80.64
N$117
  Bottom 1.27: X33.5 118.75,74.93 118.75,68.12 K6.P2
N$118
  Bottom 1.27: X33.6 116.84,71.75 116.84,65.05 K6.O2
N$119
  Top 1.27: 113.67,80.64 113.67,74.93 110.49,71.75 110.49,68.88 K6.P1
  Top 2.54: X33.2 113.67,80.64
N$120
  Top 1.27: 118.75,80.64 118.75,73.66 115.8,70.71 K6.S1
  Top 2.54: X33.1 118.75,80.64
N$121
  Top 1.27: 128.91,80.64 128.91,74.93 125.73,71.75 125.73,68.88 K7.P1
  Top 2.54: X34.2 128.91,80.64
N$122
  Top 1.27: 144.15,80.64 144.15,74.93 140.97,71.75 140.97,68.88 K8.P1
  Top 2.54: X35.2 144.15,80.64
N$316
  Bottom 1.27: X35.5 149.22,74.93 149.22,68.12 K8.P2
N$317
  Bottom 1.27: X35.6 147.32,71.75 147.32,65.05 K8.O2
N$318
  Top 1.27: 108.58,80.64 108.58,65.81 K6.O1
  Top 2.54: X33.3 108.58,80.64
N$319
  Top 1.27: 139.06,80.64 139.06,65.81 K8.O1
  Top 2.54: X35.3 139.06,80.64
N$320
  Top 1.27: 123.83,80.64 123.83,65.81 K7.O1
  Top 2.54: X34.3 123.83,80.64
N$321
  Bottom 1.27: X34.6 132.08,71.75 132.08,65.05 K7.O2
N$322
  Bottom 1.27: X34.5 133.99,74.93 133.99,68.12 K7.P2
N$323
  Top 2.54: X33.4 121.28,70.84 K6.S2
N$324
  Top 2.54: X34.4 136.53,70.84 K7.S2
N$325
  Top 1.27: 133.99,80.64 133.99,76.2 133.99,75.79 133.99,73.66 131.04,70.71 K7.S1
  Top 2.54: X34.1 133.99,80.64
N$326
  Top 1.27: 149.22,80.64 149.22,73.66 146.28,70.71 K8.S1
  Top 2.54: X35.1 149.22,80.64
N$327
  Top 2.54: X35.4 151.76,70.84 K8.S2
OC_R1  (via drill 0.5)
  Top 0.305: RN2.8 89.95,24.26 88.77,24.26 88.14,23.62 IC3.11 85.8,23.5 v83.82,23.5 | K8.2 139.06,40.64 92.71,40.64 v90.81,38.73
  Bottom 0.305: v90.81,38.73 90.81,33.02 83.82,26.04 v83.82,23.5
OC_R2  (via drill 0.5)
  Top 0.305: RN2.7 89.99,25.02 88.39,25.02 88.27,24.89 IC3.12 85.8,24.77 v82.55,24.77 | v88.9,38.73 91.44,41.27 124.46,41.27 K7.2
  Bottom 0.305: v88.9,38.73 88.9,33.02 82.55,26.67 v82.55,24.77
OC_R3  (via drill 0.5)
  Top 0.305: RN2.6 89.99,25.78 88.52,25.78 88.14,26.16 IC3.13 81.53,26.16 81.41,26.04 v81.28,26.04 | K6.2 109.86,41.91 90.17,41.91 v87,38.73
  Bottom 0.305: v87,38.73 87,33.02 81.28,27.3 v81.28,26.04
OC_R4  (via drill 0.5)
  Top 0.305: RN2.5 89.94,26.67 88.9,26.67 88.14,27.43 IC3.14 85.8,27.3 v80.01,27.3 | v85.09,38.73 88.9,42.55 95.25,42.55 K5.2
  Bottom 0.305: v85.09,38.73 85.09,33.02 80.01,27.94 v80.01,27.3
OC_R5  (via drill 0.5)
  Top 0.305: RN3.4 89.94,29.21 88.9,29.21 88.39,28.7 IC3.15 85.8,28.83 79.63,28.83 v79.38,28.57 | v83.19,38.73 80.26,41.66 70.1,41.66 K4.2
  Bottom 0.305: v83.19,38.73 83.19,32.39 v79.38,28.57
OC_R6  (via drill 0.5)
  Top 0.305: RN3.3 89.9,29.97 IC3.16 85.8,30.1 79.63,30.1 79.38,29.84 v78.74,29.84 | v81.28,38.73 79.38,40.64 66.04,40.64 65.41,41.27 65.41,43.18 64.77,43.81 52.7,43.81 K3.2
  Bottom 0.305: v81.28,38.73 81.28,31.75 79.38,29.84 v78.74,29.84
OC_R7  (via drill 0.5)
  Top 0.305: RN3.2 89.99,30.86 88.52,30.86 88.14,31.24 IC3.17 85.8,31.12 v78.11,31.12 | v79.38,38.73 78.11,40 65.41,40 64.77,40.64 64.77,42.55 64.14,43.18 35.94,43.18 35.56,43.56 K2.2
  Bottom 0.305: v79.38,38.73 79.38,34.29 80.01,33.66 80.01,31.75 79.38,31.12 v78.11,31.12
OC_R8  (via drill 0.5)
  Top 0.305: RN3.1 89.95,31.62 88.9,31.62 88.01,32.51 IC3.18 84.2,32.51 84.07,32.39 v78.74,32.39 | v77.47,38.73 65.41,38.73 64.14,40 64.14,41.91 63.5,42.55 21.34,42.55 20.32,43.56 K1.2
  Bottom 0.305: v77.47,38.73 77.47,34.29 v78.74,32.39
REG_5V  (via drill 0.5, 0.9)
  Top 0.254: RN6.6 RN6.5 47.23,29.59 47.75,29.59 48.13,29.97 v48.51,29.97 | 44.98,24.41 45.09,24.51
  Top 0.305: R1.A 102.35,38.85 102.87,39.37 107.95,39.37 | 107.95,39.37 113.67,39.37 | 113.67,39.37 119.38,39.37 | 119.38,39.37 125.09,39.37 | 125.09,39.37 130.81,39.37 | 130.81,39.37 136.53,39.37 | 136.53,39.37 141.6,39.37 142.24,38.73 142.24,37.58 R8.A | R7.A 136.64,39.25 136.53,39.37 | R6.A 130.93,39.25 130.81,39.37 | R5.A 125.21,39.25 125.09,39.37 | R4.A 119.5,39.25 119.38,39.37 | R3.A 113.78,39.25 113.67,39.37 | R2.A 108.06,39.25 107.95,39.37 | H1.1 7.46,19.27 4.95,16.76 4.95,15.83 RNB.6
  Top 0.406: U$18.A3 U$18.A2 U$18.A1 | IC2.18 70.36,32.51 69.85,33.02 69.85,36.47 CB3.2 CA3.2 67.29,34.9 v66.67,34.29 67.94,33.02 67.94,30.86 65.41,28.32 65.41,27.3 64.26,26.16 IC2.6 62.71,26.04 | v1.91,18.41 4.45,20.95 7.37,20.95 H1.1
  Top 0.61: 69.22,37.11 CB3.2 | FOR_NANO.5V 57.78,31.75 58.42,31.12 58.42,27.56 59.82,26.16 IC2.6 | v48.51,29.97 48.51,28.19 45.09,24.77 45.09,24.51 X1.2
  Top 0.813: IC2.18 73.15,32.51 73.66,33.02 73.66,33.66 74.3,34.29 88.9,34.29 93.34,38.73 97.16,38.73 | 97.16,38.73 102.23,38.73 102.35,38.85 | C1.+ 96.77,38.35 97.16,38.73 | 16.13,20.83 9.96,20.83 H1.1 | 16.13,20.83 17.27,20.83 18.41,19.69 20.75,19.69 C4.1 | IC1.4 16.13,19.15 16.13,20.83
  Top 1.016: H1.1 9.27,18.41 9.27,17.65 9.4,17.53 9.4,5.59 13.46,1.52 37.72,1.52 38.73,2.54 38.73,6.35 39.37,6.99 44.83,6.99 v45.09,7.24 45.21,7.37 | 22.05,19.69 22.23,19.69 22.86,20.32 22.86,26.67 v20.32,29.21
  Top 1.27: 20.75,19.69 22.05,19.69
  Bottom 0.254: U$18.A3 3.17,25.4 1.91,24.13 v1.91,18.41
  Bottom 0.61: FOR_NANO.5V 50.29,31.75 v48.51,29.97
  Bottom 1.016: v45.09,7.24 X1.2
REG_12V  (via drill 0.5)
  Top 0.61: IC1.7 13.46,23.16 | 14.1,22.48 14.15,22.48
  Top 0.813: v18.41,22.48 14.15,22.48 13.46,23.16 | v25.4,22.48 26.04,21.84 C3.1 26.04,14.61 27.3,13.34 BRA1.+
  Bottom 0.813: v18.41,22.48 v25.4,22.48
UNREG_12V  (via drill 0.5, 0.9)
  Top 0.762: v95.38,22.35 IC3.10
  Top 2.54: X2.2 26.97,7.32 21.59,12.7 BRA1.~@1 21.59,15.24 | 21.59,15.24 BRA1.~@2 | U$1.TIP 15.14,13.87 16.51,15.24 21.59,15.24
  Bottom 1.016: C2.+ 85.72,41.91
  Bottom 1.27: 98.81,41.91 98.81,25.78 v95.38,22.35
  Bottom 1.422: v27.94,31.75 27.94,41.91
  Bottom 1.778: 43.18,41.91 27.94,41.91 27.81,41.91 K1.1 | 73.66,41.91 58.42,41.91 | 58.42,41.91 43.18,41.91 | 43.18,41.91 43.18,45.59 K2.1 | K3.1 58.29,42.04 58.42,41.91 | 106.05,41.91 98.81,41.91 85.72,41.91 73.66,41.91 | 106.05,41.91 120.65,41.91 | 120.65,41.91 136.53,41.91 | 136.53,41.91 151.13,41.91 151.76,42.55 151.76,45.59 K8.1 | K7.1 136.4,42.04 136.53,41.91 | K6.1 121.16,42.42 120.65,41.91 | K5.1 105.92,42.04 106.05,41.91 | 73.66,41.91 73.66,45.59 K4.1 73.53,42.04 73.66,41.91 | v27.94,31.75 27.94,5.44 X2.2

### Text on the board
tNames: 1 | 8 | 4 | 5 | Bank 1 | A0 | A1 | A2 | Address | SC | SCL | SDA | 5V | GND | 2016 ControlEverything.com | MCP23008 | ANSR8xDPDT | REV.E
